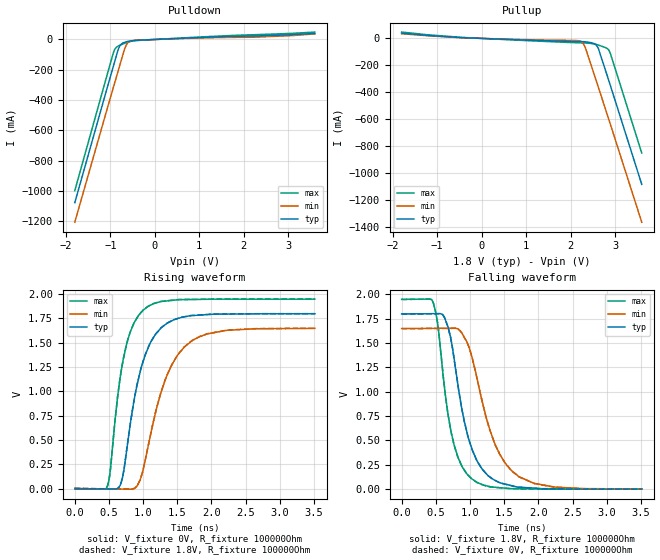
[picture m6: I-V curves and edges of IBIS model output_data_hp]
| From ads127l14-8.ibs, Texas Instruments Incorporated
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|   output_data_hp Model
[Model]   output_data_hp
Model_type   Output
Polarity   Non-Inverting
Vmeas = 0.9
Vref = 0
Cref = 2pF
Rref = 100000
|   typ   min   max
C_comp   0.609pF   0.629pF   0.591pF
[Voltage Range]   1.8   1.65   1.95
[Temperature Range]   27   125   -40
[Pullup Reference]   1.8   1.65   1.95
[Pulldown Reference]   0   0   0
[Power Clamp Reference]   1.8   1.65   1.95
[GND Clamp Reference]   0   0   0
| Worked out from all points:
|   slope of the pulldown table from 0 to 0.27 V, typ, clamps not added: 75.1 ohm
|   slope of the pullup table from 0 to 0.27 V, typ, clamps not added: 77.9 ohm
|   falling waveform, V_fixture 1.8V, R_fixture 100000Ohm: 20-80 % time 313ps typ, 417ps min, 245ps max; typ from 1.8 V to 0.001 V
|   rising waveform, V_fixture 0V, R_fixture 100000Ohm: 20-80 % time 316ps typ, 417ps min, 241ps max; typ from 0 V to 1.8 V
|   rising waveform, V_fixture 1.8V, R_fixture 100000Ohm: 20-80 % time 316ps typ, 416ps min, 240ps max; typ from 0.001 V to 1.8 V
|   falling waveform, V_fixture 0V, R_fixture 100000Ohm: 20-80 % time 313ps typ, 417ps min, 245ps max; typ from 1.8 V to 0 V
[Pulldown]
|   Voltage   I(typ)   I(min)   I(max)
-1.8V     -1.077A    -1.205A    -997.2mA
-1.071V   -318.9mA   -456.6mA   -231.7mA
-914.4mV  -157.9mA   -298.1mA   -73.53mA
-871.2mV  -114mA     -254.4mA   -52.93mA
-817.2mV  -61.41mA   -199.9mA   -42.56mA
-774mV    -36.14mA   -156.4mA   -36.81mA
-671.4mV  -17.91mA   -56.11mA   -24.35mA
-639mV    -15.26mA   -34.55mA   -20.85mA
-590.4mV  -11.99mA   -16.69mA   -16.22mA
-369mV    -4.99mA    -4.05mA    -6.211mA
2.261V    22.91mA    15.45mA    31.55mA
3.6V      39.88mA    36.83mA    48.75mA
[Pullup]
|   Voltage   I(typ)   I(min)   I(max)
-1.8V     39mA       34.48mA    46.78mA
-444.6mV  5.876mA    4.778mA    7.406mA
2.093V    -22.41mA   -15.07mA   -31.52mA
2.25V     -23.54mA   -26.56mA   -33.34mA
2.326V    -25.06mA   -64.32mA   -34.2mA
2.531V    -38.47mA   -267.6mA   -41.03mA
2.585V    -51.83mA   -322.1mA   -45.36mA
2.628V    -78.48mA   -365.7mA   -49.53mA
2.812V    -263.9mA   -551.8mA   -72.05mA
2.871V    -325mA     -612.3mA   -93.68mA
2.984V    -442.1mA   -728.3mA   -204.8mA
3.6V      -1.081A    -1.361A    -848.7mA
[Ramp]
R_load = 100000
|   typ   min   max
dV/dt_r   1.07917/3.12946e-10   0.989044/4.12093e-10   1.16929/2.40102e-10
dV/dt_f   1.0792/3.10526e-10   0.989082/4.14531e-10   1.1693/2.42665e-10
[Falling Waveform]
V_fixture = 1.8V
V_fixture_min = 1.65V
V_fixture_max = 1.95V
R_fixture = 100000Ohm
C_fixture = 0F
|   Time   V(typ)   V(min)   V(max)
0s        1.8V       1.65V      1.95V
459.5ps   1.803V     1.652V     1.921V
525.2ps   1.803V     1.652V     1.71V
617.6ps   1.776V     1.653V     1.101V
767.7ps   1.338V     1.654V     453.5mV
885.5ps   805.4mV    1.599V     230.3mV
1.022ns   426.1mV    1.374V     108.3mV
1.356ns   94.24mV    479.7mV    20.03mV
1.709ns   20.95mV    132mV      4.583mV
3.512ns   1.43mV     1.714mV    1.195mV
[Rising Waveform]
V_fixture = 0V
V_fixture_min = 0V
V_fixture_max = 0V
R_fixture = 100000Ohm
C_fixture = 0F
|   Time   V(typ)   V(min)   V(max)
0s        5.563nV    56.21nV    55.5nV
477.9ps   -3.564mV   -3.169mV   26.38mV
521.8ps   -3.892mV   -3.461mV   201.7mV
638.1ps   5.22mV     -4.232mV   1.008V
711.5ps   164.5mV    -4.718mV   1.338V
873.5ps   933mV      2.05mV     1.712V
1.001ns   1.311V     196.1mV    1.836V
1.322ns   1.686V     1.116V     1.929V
1.709ns   1.78V      1.518V     1.945V
3.512ns   1.799V     1.648V     1.949V
[Rising Waveform]
V_fixture = 1.8V
V_fixture_min = 1.65V
V_fixture_max = 1.95V
R_fixture = 100000Ohm
C_fixture = 0F
|   Time   V(typ)   V(min)   V(max)
0s        1.332mV    1.528mV    1.161mV
477.9ps   -2.208mV   -1.603mV   27.61mV
521.8ps   -2.534mV   -1.891mV   203mV
638.1ps   6.634mV    -2.653mV   1.01V
711.5ps   166.1mV    -3.133mV   1.34V
873.5ps   934.8mV    3.718mV    1.713V
1.001ns   1.313V     198.2mV    1.837V
1.322ns   1.687V     1.118V     1.93V
1.709ns   1.781V     1.52V      1.947V
3.512ns   1.8V       1.65V      1.95V
[Falling Waveform]
|Gnd
V_fixture = 0V
V_fixture_min = 0V
V_fixture_max = 0V
R_fixture = 100000Ohm
C_fixture = 0F
|   Time   V(typ)   V(min)   V(max)
0s        1.799V     1.648V     1.949V
459.5ps   1.802V     1.651V     1.92V
525.2ps   1.802V     1.651V     1.708V
617.6ps   1.775V     1.651V     1.1V
767.7ps   1.336V     1.652V     452.1mV
885.5ps   803.5mV    1.597V     229.1mV
1.022ns   424.5mV    1.372V     107.1mV
1.356ns   92.84mV    477.5mV    18.86mV
1.709ns   19.6mV     130.3mV    3.421mV
3.512ns   98.34uV    186.1uV    34.58uV
